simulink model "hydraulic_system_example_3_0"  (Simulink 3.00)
settings: Solver=ode23  StartTime=0.0  StopTime=5  MaxStep=0.01  RelTol=1e-3
StopFcn:
  | Final1
undefined symbols (not defined in the file or in its folder): Final, l, m3, s, to
libraries: simulink3 x2

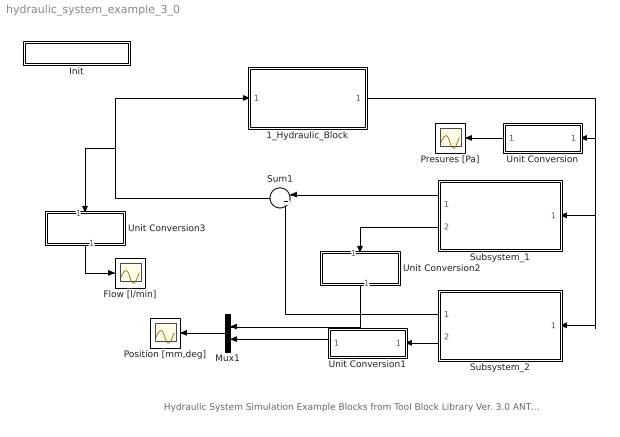
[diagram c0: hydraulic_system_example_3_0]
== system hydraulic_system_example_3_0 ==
  note: Hydraulic System Simulation Example Blocks from Tool Block Library Ver. 3.0 ANTEA s.a.s.
  1_Hydraulic_Block : Subsystem
  Flow [l/min] : Scope
  Init : Subsystem  mask(Initialisation){Name_in=Final, Name_fin=Final, Ch=Unitialised Condition, Sav=off}
      mask prompts: Name_in "Initial state File Name"; Name_fin "Final state File Name"; Ch "Start from"; Sav "Save Current States to File"
      mask init:
      | global nome_f
      | global nome_i
      | 
      | 
      | if Ch==2
      |   set_param(gcs,'SaveFinalState','on')
      |   set_param(gcs,'FinalStateName','x_Final')
      |   set_param(gcs,'LoadInitialState','on')
      |   set_param(gcs,'InitialState','x_Final')
      | end
      | if Ch==3
      |   set_param(gcs,'LoadInitialState','off')
      |   set_param(gcs,'SaveFinalState','on')
      |   set_param(gcs,'FinalStateName','x_Final')
      | end
      | if Ch==1
      |   nome_i = Name_in;
      |     set_param(gcs,'InitialState','x_Initial')
      |     set_param(gcs,'LoadInitialState','on')
      |     set_param(gcs,'SaveFinalState','on')
      |     set_param(gcs,'FinalStateName','x_Final')
      |     run start_r
      | end
      | 
      | if Sav==1
      |   nome_f = Name_fin;
      |   set_param(gcs,'StopFcn','Initial1')
      | else
      |   set_param(gcs,'StopFcn','Final1')
      | end
  Mux1 : Mux  Orientation=left  Inputs=2
  Position [mm,deg] : Scope
  Presures [Pa] : Scope
  Subsystem_1 : Subsystem  Orientation=left
  Subsystem_2 : Subsystem  Orientation=left
  Sum1 : Sum  Orientation=left  Inputs=|++  SaturateOnIntegerOverflow=on
  Unit Conversion : Subsystem  Orientation=left  mask(Unit conversion){Ch=Pa to MPa}
      mask prompts: Ch "Conversion type"
      mask init:
      | if Ch==1
      |   gain = 6e4;
      |  dsp = 'm3/s to l/min';
      | end
      | if Ch==2
      |   gain = 6.102e4;
      |   dsp = 'm3/s to cis';
      | end
      | if Ch==3
      |   gain = 15852;
      |   dsp = 'm3/s to gpm';
      | end
      | if Ch==4
      |   gain = 1e-6;
      |   dsp = 'Pa to MPa';
      | end
      | if Ch==5
      |   gain = 1.4503e-4;
      |   dsp = 'Pa to psi';
      | end
      | if Ch==6
      |   gain = 1000;
      |   dsp = 'm to mm';
      | end
      | if Ch==7
      |   gain = 39.37;
      |   dsp = 'm to in';
      | end
      | if Ch==8
      |   gain = 180/pi;
      |   dsp = 'rad to deg';
      | end
  Unit Conversion1 : Subsystem  Orientation=left  mask(Unit conversion){Ch=rad to deg}
      mask prompts: Ch "Conversion type"
      mask init:
      | if Ch==1
      |   gain = 6e4;
      |  dsp = 'm3/s to l/min';
      | end
      | if Ch==2
      |   gain = 6.102e4;
      |   dsp = 'm3/s to cis';
      | end
      | if Ch==3
      |   gain = 15852;
      |   dsp = 'm3/s to gpm';
      | end
      | if Ch==4
      |   gain = 1e-6;
      |   dsp = 'Pa to MPa';
      | end
      | if Ch==5
      |   gain = 1.4503e-4;
      |   dsp = 'Pa to psi';
      | end
      | if Ch==6
      |   gain = 1000;
      |   dsp = 'm to mm';
      | end
      | if Ch==7
      |   gain = 39.37;
      |   dsp = 'm to in';
      | end
      | if Ch==8
      |   gain = 180/pi;
      |   dsp = 'rad to deg';
      | end
      | gain=1;
  Unit Conversion2 : Subsystem  Orientation=down  mask(Unit conversion){Ch=m to mm}
      mask prompts: Ch "Conversion type"
      mask init:
      | if Ch==1
      |   gain = 6e4;
      |  dsp = 'm3/s to l/min';
      | end
      | if Ch==2
      |   gain = 6.102e4;
      |   dsp = 'm3/s to cis';
      | end
      | if Ch==3
      |   gain = 15852;
      |   dsp = 'm3/s to gpm';
      | end
      | if Ch==4
      |   gain = 1e-6;
      |   dsp = 'Pa to MPa';
      | end
      | if Ch==5
      |   gain = 1.4503e-4;
      |   dsp = 'Pa to psi';
      | end
      | if Ch==6
      |   gain = 1000;
      |   dsp = 'm to mm';
      | end
      | if Ch==7
      |   gain = 39.37;
      |   dsp = 'm to in';
      | end
      | if Ch==8
      |   gain = 180/pi;
      |   dsp = 'rad to deg';
      | end
      | gain=1;
  Unit Conversion3 : Subsystem  Orientation=down  mask(Unit conversion){Ch=m3/s to l/min}
      mask prompts: Ch "Conversion type"
      mask init:
      | if Ch==1
      |   gain = 6e4;
      |  dsp = 'm3/s to l/min';
      | end
      | if Ch==2
      |   gain = 6.102e4;
      |   dsp = 'm3/s to cis';
      | end
      | if Ch==3
      |   gain = 15852;
      |   dsp = 'm3/s to gpm';
      | end
      | if Ch==4
      |   gain = 1e-6;
      |   dsp = 'Pa to MPa';
      | end
      | if Ch==5
      |   gain = 1.4503e-4;
      |   dsp = 'Pa to psi';
      | end
      | if Ch==6
      |   gain = 1000;
      |   dsp = 'm to mm';
      | end
      | if Ch==7
      |   gain = 39.37;
      |   dsp = 'm to in';
      | end
      | if Ch==8
      |   gain = 180/pi;
      |   dsp = 'rad to deg';
      | end
      | gain=1;
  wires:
  Subsystem_1/1(Valve Flow) -> Sum1/1
  Mux1/1 -> Position [mm,deg]/1
  1_Hydraulic_Block/1(Pressures) -> Subsystem_2/1(Pressures), Subsystem_1/1(Pressures), Unit Conversion/1(Input)
  Sum1/1 -> 1_Hydraulic_Block/1(Valve Flows), Unit Conversion3/1(Input)
  Unit Conversion/1(Out1) -> Presures [Pa]/1
  Subsystem_2/1(Valve Flow) -> Sum1/2
  Unit Conversion2/1(Out1) -> Mux1/1
  Subsystem_1/2(Actuator Position) -> Unit Conversion2/1(Input)
  Unit Conversion1/1(Out1) -> Mux1/2
  Subsystem_2/2(Actuator Position) -> Unit Conversion1/1(Input)
  Unit Conversion3/1(Out1) -> Flow [l/min]/1

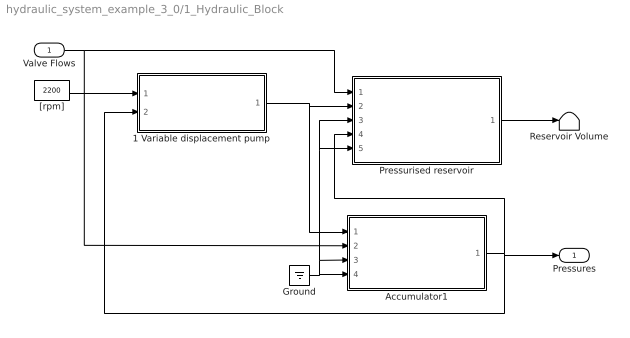
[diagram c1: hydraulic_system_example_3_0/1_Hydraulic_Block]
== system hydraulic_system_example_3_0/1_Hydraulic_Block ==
  Valve Flows : Inport  Port=1  PortWidth=-1  SampleTime=-1  DataType=auto
  1 Variable displacement pump : Subsystem  mask(Variable Displacement Pump){deltax=15.5, deltamn=0, pm_min=18, pm_max=20, tau=.005, eta_m=.95, eta_vol=.95, rho_e=800, mu_e=.002, beta_e=730}
      mask prompts: deltax "Pump max displacement [cc/rev]"; deltamn "Pump min displacement [cc/rev]"; pm_min "Minimum compensation pressure [MPa]"; pm_max "Maximum compensation pressure [MPa]"; tau "Compensator time constant [s]"; eta_m "Mechanical efficiency"; eta_vol "Volumetric efficiency"; rho_e "Fluid density [kg/m3]"; mu_e "Fluid viscosity [kg/ms]"; beta_e "Bulk modulus [MPa]"
      mask help: Model of a variable displacement pump.
      mask init:
      | global rho
      | global mu
      | global beta
      | rho=rho_e;
      | mu=mu_e;
      | beta=beta_e*1e6;
      | dlt_max=deltax*1e-6/60;
      | dlt_min=deltamn*1e-6/60;
      | p_max = pm_max*1.e6;
      | p_min = pm_min*1.e6;
  Accumulator1 : Subsystem  mask(Accumulator){ti=20, Tp=20, cv=742, h_gas=.2, hy_compl=4e-14, vi=.3, pp=12, r_gas=297}
      mask prompts: ti "Initial liquid temperature [°C]"; Tp "Precharge temperature [°C]"; cv "Gas specific heat (cv) [J/(K kg)]"; h_gas "Heat exchange coefficient [W/K]"; hy_compl "Hydraulic compliance (with acc. discharged)[m5/N]"; vi "Precharge volume [l]"; pp "Precharge pressure [MPa]"; r_gas "Gas constant [J/(kg K)]"
      mask help: Model of a hydraulic accumulator.
      mask init:
      | global rho
      | 
      | t_liq = ti+273;
      | t_pr = Tp+273;
      | T0 = t_liq;
      | P0 = pp*1e6;
      | v0=vi/1000;
      | m_gas=P0*v0/(r_gas*t_pr);
      | P0 = pp*1e6*T0/t_pr;
  Ground : Ground
  Pressurised reservoir : Subsystem  mask(Pressurised Reservoir){v_cc=200, a_hp=0.0001, a_lp=0.0067, k_spr_res=0, f0_res=0}
      mask prompts: v_cc "Initial fluid volume [cc]"; a_hp "High pressure side area [m2]"; a_lp "Low pressure side area  [m2]"; k_spr_res "Spring stiffness [N/m]"; f0_res "Spring preload [N]"
      mask help: Model of a pressurised reservoir;
      mask init:
      | v_reser=v_cc/1e6;
  Reservoir Volume : Terminator
  "[rpm]" : Constant  Value=2200
  Pressures : Outport  Port=1  InitialOutput=0
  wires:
  "[rpm]"/1 -> 1 Variable displacement pump/1(Angular speed)
  Valve Flows/1 -> Pressurised reservoir/1(Out _Flows), Accumulator1/2(Out_Flow)
  Accumulator1/1(Out_Pressures) -> Pressurised reservoir/4(Pressures), Pressures/1, 1 Variable displacement pump/2(Pressure)
  Pressurised reservoir/1(Reservoir volume) -> Reservoir Volume/1
  1 Variable displacement pump/1(Pump flow) -> Accumulator1/1(Pump flow), Pressurised reservoir/2(Pump flow)
  Ground/1 -> Accumulator1/4(Single acting act. unctrl. flow), Accumulator1/3(Relief flow), Pressurised reservoir/5(Single acting act. unctrl. flow), Pressurised reservoir/3(Relief flow)

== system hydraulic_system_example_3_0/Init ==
  Subsystem : Subsystem

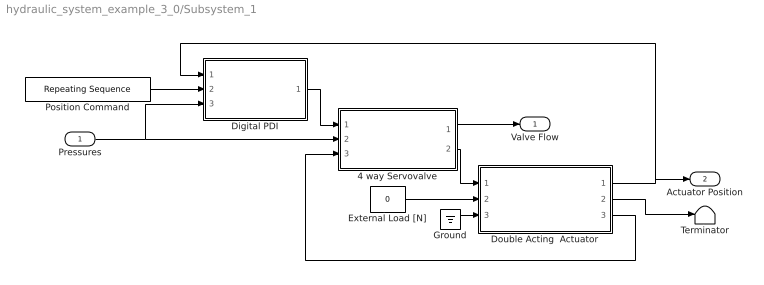
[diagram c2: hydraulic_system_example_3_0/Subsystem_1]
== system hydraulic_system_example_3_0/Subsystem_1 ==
  Pressures : Inport  Port=1  PortWidth=-1  SampleTime=-1  DataType=auto
  4 way Servovalve : Subsystem
  Digital PDI : Subsystem  mask(PDI controller){Ts=3.e-2, Tc=1.e-2, Gp=[0.1 0.1], Gi=[0 0], Gd=[0 0], tau=0, Ls=[0 0], Ls_1=[-Inf Inf], i_i_max=[-Inf Inf], H=1000, p_opm=16, max_cp=Inf, max_cm=-Inf}
      mask prompts: Ts "Sampling time [s]"; Tc "Calculation time [s]"; Gp "Proportional gain (2 values: [- +])"; Gi "Integrative gain (2 values: [- +])"; Gd "Derivative gain (2 values: [- +])"; tau "First order filter constant [s]"; Ls "Integrator threshold (2 values)"; Ls_1 "Integrator band limit (2 values)"; i_i_max "Integrator current saturation [mA] (2 val)"; H "Feedback gain"; p_opm "Minimum Operative Pressure [MPa]"; max_cp "max curr"; max_cm "min curr"
      mask help: Digital PDI controller
      mask init:
      | % i_i_min=-i_i_max;
      | % Li=-Ls;
      | % Li_1=-Ls_1;
      | p_op=p_opm*1.e6;
  Double Acting  Actuator : Subsystem  mask{Ai=1.13e-4, Au=0.38e-4, X_s=[0 0.05], m=0.5, V0_out=1.5e-5, V0_in=1.5e-5, F0=0, K=0, C=1, c_leak=0, Fs=1, Fd=1}
      mask prompts: Ai "Piston Input Area [m2]"; Au "Piston Output Area [m2]"; X_s "Piston Maximum Stroke [m]"; m "Piston Mass [kg]"; V0_out "Piston Outlet Lost Volume [m3]"; V0_in "Piston Inlet Lost Volume [m3]"; F0 "Piston Spring Preload [N]"; K "Piston Spring Stiffness [N/m]"; C "Piston Damping [N/(m/s)]"; c_leak "Piston leakage coefficient [(m3/s)/sqr(Pa)]"; Fs "Static Friction Force [N]"; Fd "Dynamic Friction Force [N]"
      mask init:
      | global beta
  External Load [N] : Constant  Value=0
  Ground : Ground
  Position Command : simulink3/Sources/Repeating Sequence  rep_seq_t="[0     .5   .5     1.5    1.5    2.5]"  rep_seq_y="[0    0    40     40     20     20]"
  Terminator : Terminator
  Valve Flow : Outport  Port=1
  Actuator Position : Outport  Port=2
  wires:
  4 way Servovalve/1(In_Flows) -> Valve Flow/1
  4 way Servovalve/2(Out_Flows) -> Double Acting  Actuator/1(In_Flows)
  Pressures/1 -> Digital PDI/3(Pressures), 4 way Servovalve/2(In_Pressures)
  External Load [N]/1 -> Double Acting  Actuator/2(F_ext)
  Digital PDI/1(Current) -> 4 way Servovalve/1(Curr)
  Double Acting  Actuator/1(Position) -> Actuator Position/1, Digital PDI/1(Feedback)
  Position Command/1 -> Digital PDI/2(Demand)
  Double Acting  Actuator/3(In_pressures) -> 4 way Servovalve/3(Out_Pressures)
  Double Acting  Actuator/2("Speed ") -> Terminator/1
  Ground/1 -> Double Acting  Actuator/3(Connection load)

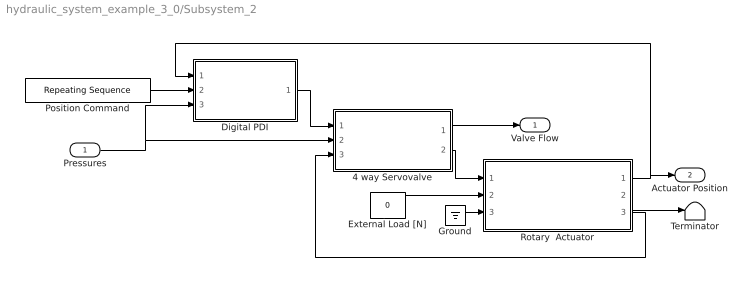
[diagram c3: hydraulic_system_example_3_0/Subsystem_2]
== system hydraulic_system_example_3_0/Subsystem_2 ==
  Pressures : Inport  Port=1  PortWidth=-1  SampleTime=-1  DataType=auto
  4 way Servovalve : Subsystem
  Digital PDI : Subsystem  mask(PDI controller){Ts=3.e-2, Tc=1.e-2, Gp=[0.01 0.005], Gi=[0 0], Gd=[0 0], tau=0, Ls=[0 0], Ls_1=[-Inf Inf], i_i_max=[-Inf Inf], H=57.3, p_opm=16, max_cp=Inf, max_cm=-Inf}
      mask prompts: Ts "Sampling time [s]"; Tc "Calculation time [s]"; Gp "Proportional gain (2 values: [- +])"; Gi "Integrative gain (2 values: [- +])"; Gd "Derivative gain (2 values: [- +])"; tau "First order filter constant [s]"; Ls "Integrator threshold (2 values)"; Ls_1 "Integrator band limit (2 values)"; i_i_max "Integrator current saturation [mA] (2 val)"; H "Feedback gain"; p_opm "Minimum Operative Pressure [MPa]"; max_cp "max curr"; max_cm "min curr"
      mask help: Digital PDI controller
      mask init:
      | % i_i_min=-i_i_max;
      | % Li=-Ls;
      | % Li_1=-Ls_1;
      | p_op=p_opm*1.e6;
  External Load [N] : Constant  Value=0
  Ground : Ground
  Position Command : simulink3/Sources/Repeating Sequence  rep_seq_t="[0     .5   .5     1.5    1.5    2.5]"  rep_seq_y="[0    0    60     60     30     30]"
  Rotary  Actuator : Subsystem  mask(Rotary Actuator){Air=1.78, X_s=[0 1.222], m=1.e-5, V0_out=1.e-5, F0=0, K=0, C=1, c_leak=0, Fs=.15, Fd=.1}
      mask prompts: Air "Displacement [cc/rev]"; X_s "Actuator Maximum Stroke [rad]"; m "Total Actuator Inertia [kg*m2]"; V0_out "Minimum Hydraulic Volume [m3]"; F0 "Actuator Spring Preload [Nm]"; K "Actuator Spring Stiffness [Nm/rad]"; C "Actuator Internal Damping [Nm/(rad/s)]"; c_leak "Actuator Internal Leakage Coefficient [(m3/s)/sqr(Pa)]"; Fs "Static Friction Force [N]"; Fd "Dynamic Friction Force [N]"
      mask init:
      | global beta
      | 
      | Ai = Air*1.e-6/6.2831853;
      | V0_in = V0_out;
      | Au = Ai;
  Terminator : Terminator
  Valve Flow : Outport  Port=1
  Actuator Position : Outport  Port=2
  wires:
  Position Command/1 -> Digital PDI/2(Demand)
  Digital PDI/1(Current) -> 4 way Servovalve/1(Curr)
  Pressures/1 -> 4 way Servovalve/2(In_Pressures), Digital PDI/3(Pressures)
  4 way Servovalve/2(Out_Flows) -> Rotary  Actuator/1(In_Flows)
  4 way Servovalve/1(In_Flows) -> Valve Flow/1
  External Load [N]/1 -> Rotary  Actuator/2("T_ext ")
  Rotary  Actuator/3(In_Pressures) -> 4 way Servovalve/3(Out_Pressures)
  Rotary  Actuator/1(Position) -> Digital PDI/1(Feedback), Actuator Position/1
  Ground/1 -> Rotary  Actuator/3(Connection Torque)
  Rotary  Actuator/2(Speed) -> Terminator/1

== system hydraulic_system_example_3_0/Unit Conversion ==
  Input : Inport  Port=1  PortWidth=-1  SampleTime=-1  DataType=auto
  Gain : Gain  Gain=gain  SaturateOnIntegerOverflow=on
  Out1 : Outport  Port=1
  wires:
  Gain/1 -> Out1/1
  Input/1 -> Gain/1

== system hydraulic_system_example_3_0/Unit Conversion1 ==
  Input : Inport  Port=1  PortWidth=-1  SampleTime=-1  DataType=auto
  Gain : Gain  Gain=gain  SaturateOnIntegerOverflow=on
  Out1 : Outport  Port=1
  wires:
  Input/1 -> Gain/1
  Gain/1 -> Out1/1

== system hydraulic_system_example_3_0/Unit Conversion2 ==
  Input : Inport  Port=1  PortWidth=-1  SampleTime=-1  DataType=auto
  Gain : Gain  Gain=gain  SaturateOnIntegerOverflow=on
  Out1 : Outport  Port=1
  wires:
  Gain/1 -> Out1/1
  Input/1 -> Gain/1

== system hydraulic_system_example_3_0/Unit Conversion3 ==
  Input : Inport  Port=1  PortWidth=-1  SampleTime=-1  DataType=auto
  Gain : Gain  Gain=gain  SaturateOnIntegerOverflow=on
  Out1 : Outport  Port=1
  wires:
  Input/1 -> Gain/1
  Gain/1 -> Out1/1

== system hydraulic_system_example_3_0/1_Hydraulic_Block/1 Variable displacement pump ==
  Angular speed : Inport  Port=1  PortWidth=-1  SampleTime=-1  DataType=auto
  Pressure : Inport  Port=2  PortWidth=-1  SampleTime=-1  DataType=auto
  Pump flow : Outport  Port=1
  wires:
  Pressure/1 -> ?

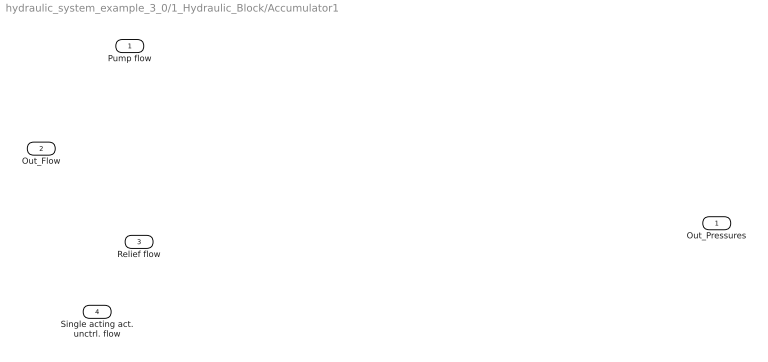
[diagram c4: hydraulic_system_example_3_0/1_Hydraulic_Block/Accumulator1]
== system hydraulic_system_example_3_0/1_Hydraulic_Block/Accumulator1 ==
  Pump flow : Inport  Port=1  PortWidth=-1  SampleTime=-1  DataType=auto
  Out_Flow : Inport  Port=2  PortWidth=-1  SampleTime=-1  DataType=auto
  Relief flow : Inport  Port=3  PortWidth=-1  SampleTime=-1  DataType=auto
  Single acting act. unctrl. flow : Inport  Port=4  PortWidth=-1  SampleTime=-1  DataType=auto
  Out_Pressures : Outport  Port=1
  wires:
  ? -> Out_Pressures/1
  Out_Flow/1 -> ?
  Relief flow/1 -> ?

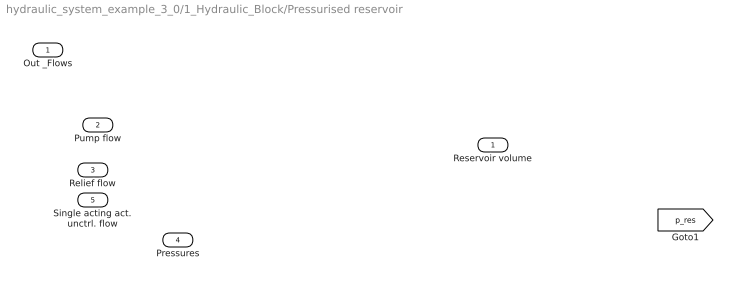
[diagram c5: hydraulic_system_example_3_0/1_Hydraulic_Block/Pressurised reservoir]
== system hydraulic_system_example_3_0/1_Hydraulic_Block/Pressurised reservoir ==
  Out _Flows : Inport  Port=1  PortWidth=-1  SampleTime=-1  DataType=auto
  Pump flow : Inport  Port=2  PortWidth=-1  SampleTime=-1  DataType=auto
  Relief flow : Inport  Port=3  PortWidth=-1  SampleTime=-1  DataType=auto
  Pressures : Inport  Port=4  PortWidth=-1  SampleTime=-1  DataType=auto
  Single acting act. unctrl. flow : Inport  Port=5  PortWidth=-1  SampleTime=-1  DataType=auto
  Reservoir volume : Outport  Port=1
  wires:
  ? -> [p_res]
  Out _Flows/1 -> ?

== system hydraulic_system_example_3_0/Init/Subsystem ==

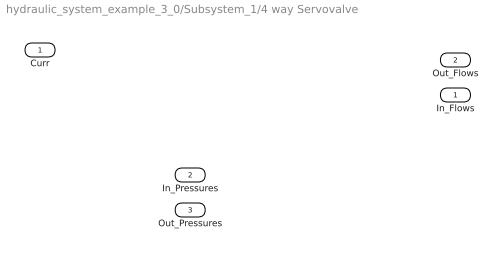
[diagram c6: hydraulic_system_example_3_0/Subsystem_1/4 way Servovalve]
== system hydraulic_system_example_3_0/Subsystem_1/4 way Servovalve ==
  Curr : Inport  Port=1  PortWidth=-1  SampleTime=-1  DataType=auto
  In_Pressures : Inport  Port=2  PortWidth=-1  SampleTime=-1  DataType=auto
  Out_Pressures : Inport  Port=3  PortWidth=-1  SampleTime=-1  DataType=auto
  In_Flows : Outport  Port=1  InitialOutput=0
  Out_Flows : Outport  Port=2  InitialOutput=0
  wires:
  ? -> In_Flows/1
  Curr/1 -> ?
  ? -> Out_Flows/1

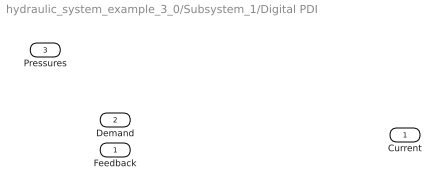
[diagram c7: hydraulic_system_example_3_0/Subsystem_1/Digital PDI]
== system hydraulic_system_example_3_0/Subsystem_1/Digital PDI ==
  Feedback : Inport  Port=1  PortWidth=-1  SampleTime=-1  DataType=auto
  Demand : Inport  Port=2  PortWidth=-1  SampleTime=-1  DataType=auto
  Pressures : Inport  Port=3  PortWidth=-1  SampleTime=-1  DataType=auto
  Current : Outport  Port=1
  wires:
  ? -> Current/1
  Pressures/1 -> ?

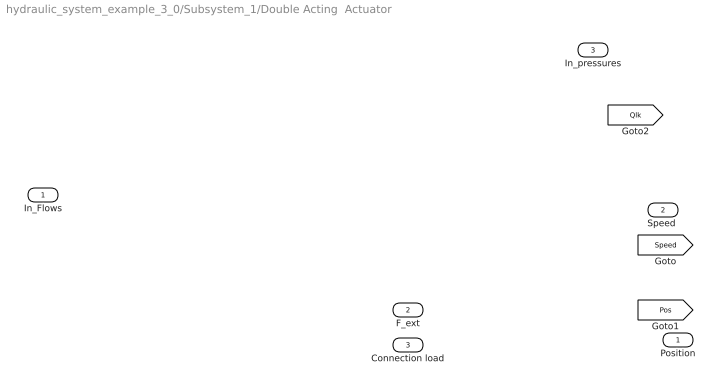
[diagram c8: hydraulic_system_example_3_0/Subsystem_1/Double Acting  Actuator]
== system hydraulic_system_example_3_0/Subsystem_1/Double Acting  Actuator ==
  In_Flows : Inport  Port=1  PortWidth=-1  SampleTime=-1  DataType=auto
  F_ext : Inport  Port=2  PortWidth=-1  SampleTime=-1  DataType=auto
  Connection load : Inport  Port=3  PortWidth=-1  SampleTime=-1  DataType=auto
  Position : Outport  Port=1
  "Speed " : Outport  Port=2
  In_pressures : Outport  Port=3
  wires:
  Connection load/1 -> ?
  F_ext/1 -> ?
  ? -> [Qlk]
  In_Flows/1 -> ?

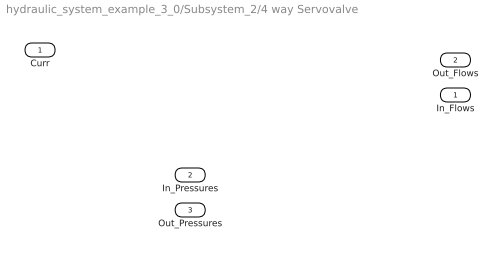
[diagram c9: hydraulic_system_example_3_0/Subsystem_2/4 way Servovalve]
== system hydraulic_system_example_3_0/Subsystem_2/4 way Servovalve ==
  Curr : Inport  Port=1  PortWidth=-1  SampleTime=-1  DataType=auto
  In_Pressures : Inport  Port=2  PortWidth=-1  SampleTime=-1  DataType=auto
  Out_Pressures : Inport  Port=3  PortWidth=-1  SampleTime=-1  DataType=auto
  In_Flows : Outport  Port=1  InitialOutput=0
  Out_Flows : Outport  Port=2  InitialOutput=0
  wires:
  ? -> In_Flows/1
  Curr/1 -> ?
  ? -> Out_Flows/1

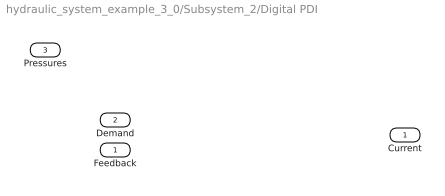
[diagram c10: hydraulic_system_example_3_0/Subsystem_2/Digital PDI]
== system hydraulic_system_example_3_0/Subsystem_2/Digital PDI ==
  Feedback : Inport  Port=1  PortWidth=-1  SampleTime=-1  DataType=auto
  Demand : Inport  Port=2  PortWidth=-1  SampleTime=-1  DataType=auto
  Pressures : Inport  Port=3  PortWidth=-1  SampleTime=-1  DataType=auto
  Current : Outport  Port=1
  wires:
  ? -> Current/1
  Pressures/1 -> ?

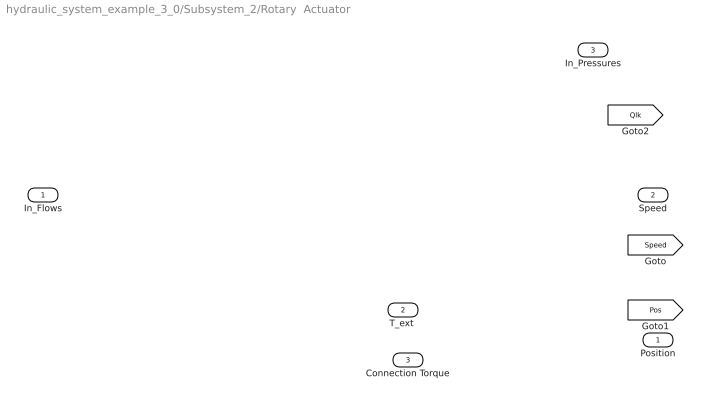
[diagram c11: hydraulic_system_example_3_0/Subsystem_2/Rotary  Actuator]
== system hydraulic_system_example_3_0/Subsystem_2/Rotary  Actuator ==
  In_Flows : Inport  Port=1  PortWidth=-1  SampleTime=-1  DataType=auto
  "T_ext " : Inport  Port=2  PortWidth=-1  SampleTime=-1  DataType=auto
  Connection Torque : Inport  Port=3  PortWidth=-1  SampleTime=-1  DataType=auto
  Position : Outport  Port=1
  Speed : Outport  Port=2
  In_Pressures : Outport  Port=3
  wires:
  ? -> Speed/1, [Speed]
  "T_ext "/1 -> ?
  Connection Torque/1 -> ?
  In_Flows/1 -> ?
  ? -> [Pos], Position/1
  ? -> [Qlk]
